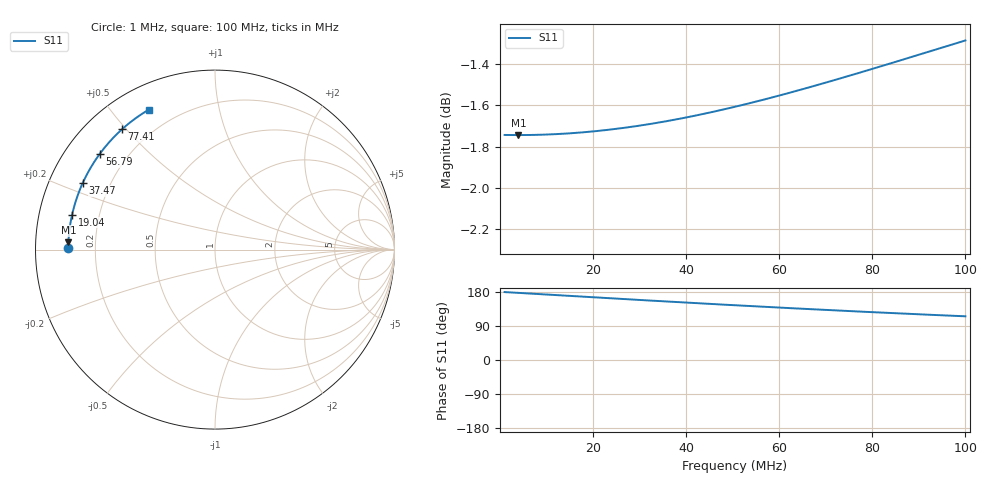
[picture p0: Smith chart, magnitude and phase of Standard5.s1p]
# MHz S RI R 50.0
! SimSmith 18.4g
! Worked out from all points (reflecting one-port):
!   1000 points, 1 MHz to 100 MHz, reference 50 ohm
!   lowest |S11| = -1.7 dB at 3.973 MHz (marker M1), VSWR 9.99, Z = 5.01 + j1.25 ohm
!   phase of S11 starts at 179 deg and turns -64 deg over the sweep
!   S11 on the Smith chart (normalised r, x): 1 MHz: 0.10, +0.01; 19.04 MHz: 0.10, +0.12; 37.47 MHz: 0.10, +0.24; 56.79 MHz: 0.10, +0.36; 77.41 MHz: 0.10, +0.49; 100 MHz: 0.10, +0.63
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1  -0.8181 0.0104
1.495496  -0.818 0.0155
3.972973  -0.817 0.0412
8.630631  -0.8133 0.0894
13.38739  -0.8069 0.1381
16.16216  -0.802 0.1663
19.03604  -0.796 0.1952
22.4054  -0.7878 0.2287
25.77478  -0.7784 0.2616
28.64865  -0.7694 0.2893
31.52252  -0.7596 0.3165
34.49549  -0.7486 0.3442
37.46847  -0.7369 0.3713
38.16216  -0.734 0.3776
44.20721  -0.7073 0.4306
50.54955  -0.6762 0.4833
56.79279  -0.6429 0.5321
62.93694  -0.6079 0.577
66.10811  -0.589 0.5989
69.18018  -0.5704 0.6193
75.32432  -0.5319 0.6577
77.40541  -0.5186 0.67
82.55856  -0.4852 0.6987
87.71171  -0.4512 0.7252
90.98198  -0.4294 0.7409
94.35135  -0.4069 0.7562
99.5045  -0.3722 0.7777
100  -0.3689 0.7797
